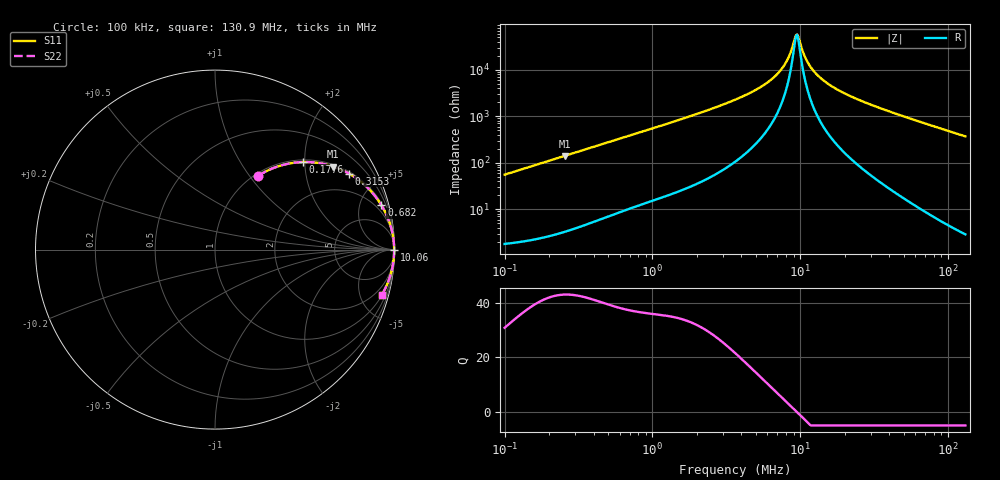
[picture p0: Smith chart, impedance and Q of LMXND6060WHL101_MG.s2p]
! LMXND6060WHL101_MG  S-PARAMETER MODEL  ( General Type )
! Model Generated by TAIYO YUDEN Corporation (http://www.ty-top.com)
! Version 1.0
! TAIYO YUDEN Control No. 191025NI43SB-FBB
! Copyright(c) 2019 TAIYO YUDEN CO.,LTD. All Rights Reserved.
! Product Description (link to TY-COMPAS)
! https://ds.yuden.co.jp/TYCOMPAS/or/detail?pn=LMXND6060WHL101MMG&u=M
! Products Name : Inductors
! Characteristics :
!  Inductance : 100 uH , SRF(min) : 3.0 MHz , DC Resistance(max) : 0.78 Ohm
!  Rated Current : Saturation :650 mA , Temp Rise : 660 mA
!  Case Size : 6.0 x 6.0 / 0.236 x 0.236 [mm/inch] , Thickness : 2.8 / 0.11 [mm/inch]
!  (Conditions: Temperature = 25 degC , DC Bias Current/Voltage = 0A / 0V)
! External Node Assignments :
!  1  o---GGG---o  2
! GND o---------o GND
! Frequency Range : 0.1MHz  -  130.914307MHz  [ 402 STEP ]
# MHz S RI R 50
! Freq[MHz].  S11 Real  S11 Imag  S21 Real  S21 Imag  S12 Real  S12 Imag  S22 Real  S22 Imag
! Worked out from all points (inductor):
!   401 points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, 100 kHz to 130.9 MHz, reference 50 ohm
!   read as one part in series: L = 88 uH near 103.7 kHz
!   highest Q = 43.1 at 254.2 kHz (marker M1), where L = 87.8 uH
!   self-resonance near 9.365 MHz
!   S11 on the Smith chart (normalised r, x): 100 kHz: 1.04, +1.11; 177.6 kHz: 1.05, +1.96; 315.3 kHz: 1.08, +3.47; 682 kHz: 1.20, +7.46; 10.06 MHz: open; 130.9 MHz: 1.06, -7.38
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0.1  0.2419 0.4124  0.7581 -0.4124  0.7581 -0.4124  0.2419 0.4124
0.177566  0.4906 0.4878  0.5094 -0.4878  0.5094 -0.4878  0.4906 0.4878
0.254219  0.6593 0.4625  0.3407 -0.4625  0.3407 -0.4625  0.6593 0.4625
0.315296  0.746 0.4237  0.254 -0.4237  0.254 -0.4237  0.746 0.4237
0.332733  0.7652 0.4123  0.2348 -0.4123  0.2348 -0.4123  0.7652 0.4123
0.682015  0.9273 0.2466  0.0727 -0.2466  0.0727 -0.2466  0.9273 0.2466
1.10711  0.9693 0.159  0.0307 -0.159  0.0307 -0.159  0.9693 0.159
3.683715  0.9961 0.0428  0.00386 -0.0428  0.00386 -0.0428  0.9961 0.0428
5.369426  0.9976 0.0235  0.00239 -0.0235  0.00239 -0.0235  0.9976 0.0235
6.902754  0.9981 0.0127  0.00193 -0.0127  0.00193 -0.0127  0.9981 0.0127
7.550657  0.9982 0.00902  0.00183 -0.00902  0.00183 -0.00902  0.9982 0.00902
8.112498  0.9982 0.00614  0.00178 -0.00614  0.00178 -0.00614  0.9982 0.00614
9.36471  0.9983 0.000481  0.00172 -0.000481  0.00172 -0.000481  0.9983 0.000481
9.706872  0.9983 -0.000929  0.00172 0.000929  0.00172 0.000929  0.9983 -0.000929
10.06153  0.9983 -0.00234  0.00172 0.00234  0.00172 0.00234  0.9983 -0.00234
10.81021  0.9983 -0.00517  0.00173 0.00517  0.00173 0.00517  0.9983 -0.00517
12.03896  0.9982 -0.00948  0.00179 0.00948  0.00179 0.00948  0.9982 -0.00948
14.40501  0.998 -0.0169  0.00198 0.0169  0.00198 0.0169  0.998 -0.0169
18.18929  0.9976 -0.0274  0.00244 0.0274  0.00244 0.0274  0.9976 -0.0274
25.1235  0.9963 -0.0446  0.00368 0.0446  0.00368 0.0446  0.9963 -0.0446
40.05754  0.9922 -0.0779  0.00782 0.0779  0.00782 0.0779  0.9922 -0.0779
130.9143  0.93 -0.2513  0.07 0.2513  0.07 0.2513  0.93 -0.2513
